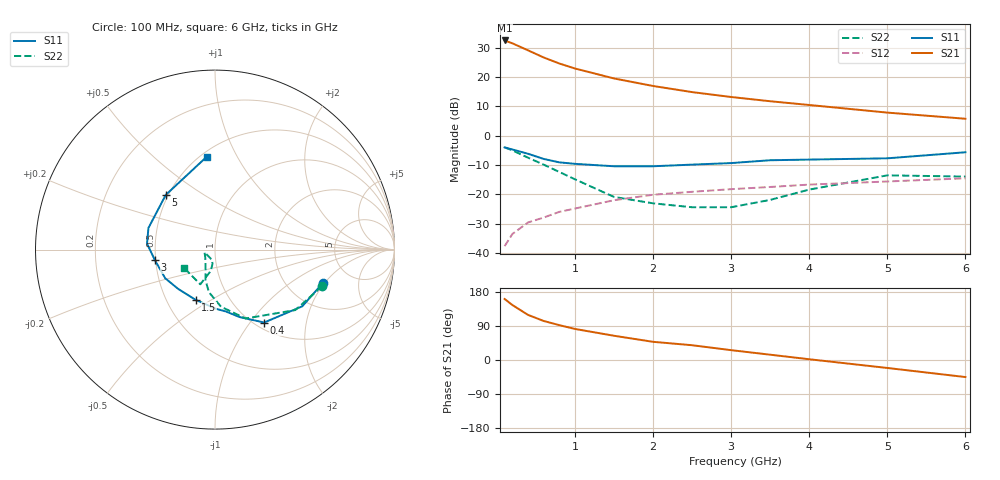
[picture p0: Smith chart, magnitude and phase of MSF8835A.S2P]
!  MSF-8835 S PARAMETERS
!  Id=36mA  LAST UPDATED 07-27-92
# ghz s ma r 50
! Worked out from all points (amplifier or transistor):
!   14 points, 100 MHz to 6 GHz, reference 50 ohm
!   highest |S21| = 32.5 dB at 100 MHz (marker M1)
!   |S21| within 3 dB of that: start of sweep to 368.8 MHz
!   unconditionally stable (mu >= 1): 2.234 GHz to end of sweep
!   at 400 MHz: K = 0.72, MSG = 29.4 dB, |S12| = -29.6 dB
!   at 2 GHz: K = 0.98, MSG = 18.6 dB, |S12| = -20.2 dB
!   at 6 GHz: K = 1.05, MAG = 8.8 dB, |S12| = -14.6 dB
!   S11 on the Smith chart (normalised r, x): 100 MHz: 3.14, -1.92; 400 MHz: 1.10, -1.17; 1.5 GHz: 0.70, -0.43; 3 GHz: 0.50, -0.07; 5 GHz: 0.48, +0.35; 6 GHz: 0.54, +0.76
0.1  0.63 -17.0  42.02 161.0  0.013 55.0  0.63 -19.0
0.2  0.58 -33.0  37.52 145.0  0.021 47.0  0.56 -37.0
0.4  0.49 -56.0  28.5 119.0  0.033 54.0  0.42 -66.0
0.6  0.4 -70.0  21.54 103.0  0.04 55.0  0.32 -84.0
0.8  0.35 -80.0  17.01 92.0  0.05 53.0  0.24 -98.0
1  0.33 -89.0  13.98 82.0  0.057 52.0  0.18 -107.0
1.5  0.3 -111.0  9.45 64.0  0.079 51.0  0.09 -126.0
2  0.3 -133.0  7.03 48.0  0.098 44.0  0.07 -141.0
2.5  0.32 -150.0  5.53 39.0  0.11 42.0  0.06 -166.0
3  0.34 -170.0  4.56 26.0  0.122 36.0  0.06 -106.0
3.5  0.38 175.0  3.86 14.0  0.133 32.0  0.08 -100.0
4  0.39 162.0  3.33 2.0  0.146 27.0  0.12 -101.0
5  0.41 132.0  2.47 -21.0  0.165 19.0  0.21 -113.0
6  0.52 95.0  1.94 -45.0  0.187 7.0  0.2 -149.0
